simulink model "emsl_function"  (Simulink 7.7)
settings: Solver=ode1  StartTime=0.0  StopTime=10.0  FixedStep=0.001  RelTol=1e-3

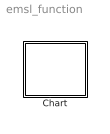
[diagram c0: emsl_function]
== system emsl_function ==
  Chart : Stateflow chart  TreatAsAtomicUnit=on

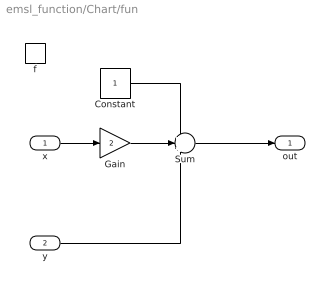
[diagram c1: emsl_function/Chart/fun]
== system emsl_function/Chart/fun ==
  x : Inport
  y : Inport  Port=2
  f : TriggerPort  TriggerType=function-call  StatesWhenEnabling=reset
  Constant : Constant
  Gain : Gain  Gain=2
  Sum : Sum  Inputs=+++
  out : Outport
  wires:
  x/1 -> Gain/1
  Gain/1 -> Sum/2
  y/1 -> Sum/3
  Constant/1 -> Sum/1
  Sum/1 -> out/1

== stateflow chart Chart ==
  state Z1
  state Z2
    en: y=fun(a,b);
  state out=fun(x,y) [function]
  Z1 -> Z2
  Z2 -> Z1
  (default) -> Z1
